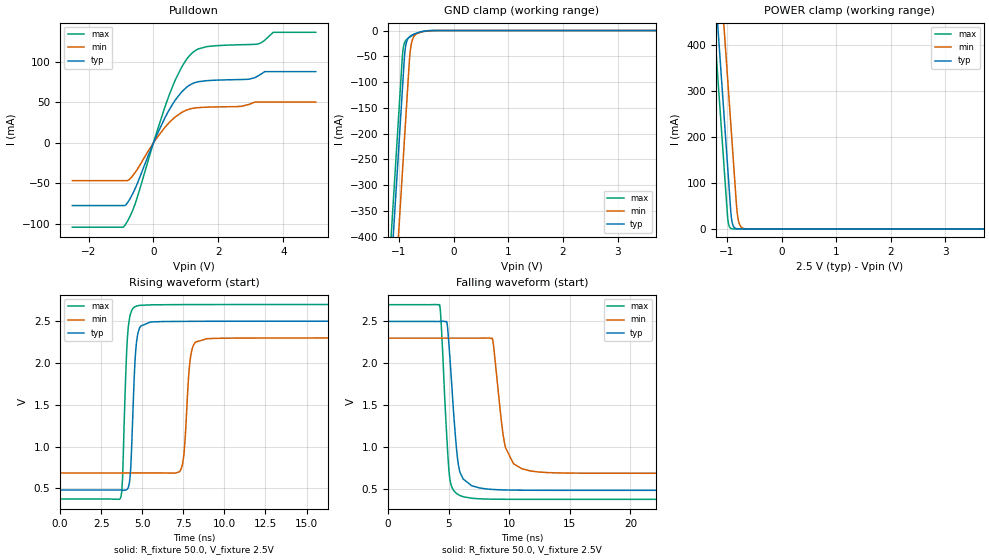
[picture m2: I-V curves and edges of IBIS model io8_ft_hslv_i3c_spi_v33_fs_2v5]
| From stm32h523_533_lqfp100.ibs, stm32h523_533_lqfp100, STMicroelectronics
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[Model]   io8_ft_hslv_i3c_spi_v33_fs_2v5
Model_type I/O_open_drain
Polarity   Non-Inverting
Enable   Active-Low
| CAP_THRESHOLD on pad IOFT is "UDTCAPC" :
| Rising=20.0% of vddiom   Falling=80.0% of vddiom
| C_comp min and max val. don't necessarily correlate with the min and max pvt
| but are the smallest and greatest pad capacitance found.
| var   typ   min   max
C_comp   3.86841pF  3.83550pF  3.96274pF
|C_comp_pulldown   3.86841pF  3.83550pF  3.96274pF
Vinl = 1.15V
Vinh = 1.35V
Vmeas = 1.25V   | Reference voltage for timing measurements
Cref  = 50.0pF   | Timing specification test load capacitance value
Rref  = 1.0MOhm   | Timing specification test load resistance value
Vref  = 1.375V   | Timing specification test load voltage
[Model Spec]
| TIME_THRESHOLD on pin ZII2CV11 is "CMOS" :
| Rising=40.0% of vdd   Falling=60.0% of vdd
Vinl 978.80000mV 906.80000mV 1.05480V
Vinh 1.39920V 1.29220V 1.48720V
| variable   typ   min   max
[Temperature Range] 25.0 125.0 -40.0
| variable   typ   min   max
[Voltage Range] 2.5V 2.3V 2.7V
| variable   typ   min   max
[POWER Clamp Reference] 2.5V 2.3V 2.7V
| variable   typ   min   max
[GND Clamp Reference] 0V 0V 0V
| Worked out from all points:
|   slope of the pulldown table from 0 to 0.375 V, typ, clamps not added: 11.5 ohm
|   GND clamp passes 1 mA (typ) near -0.52 V on its own axis
|   POWER clamp passes 1 mA (typ) near -0.84 V on its own axis
|   rising waveform, R_fixture 50.0, V_fixture 2.5V: 20-80 % time 253ps typ, 305ps min, 242ps max; typ from 0.481 V to 2.5 V
|   falling waveform, R_fixture 50.0, V_fixture 2.5V: 20-80 % time 627ps typ, 795ps min, 493ps max; typ from 2.5 V to 0.481 V
[POWER Clamp]
-2.5V     2.708A     2.899A     2.597A
-1.23V    548.8mA    740.2mA    437.5mA
-1.16V    429.8mA    621.2mA    318.5mA
-1.12V    361.8mA    553.2mA    250.5mA
-1.03V    208.8mA    400.2mA    97.53mA
-980mV    123.8mA    315.2mA    17.95mA
-920mV    26.3mA     213.2mA    906uA
-880mV    5.543mA    145.2mA    123.7uA
-810mV    363.5uA    33.6mA     3.797uA
-770mV    76.62uA    10.47mA    518.8nA
-700mV    5.026uA    1.361mA    16.09nA
5V        0A         0A         0A
[GND Clamp]
-2.5V     -2.77A     -2.931A    -2.704A
-1.21V    -576.8mA   -738.1mA   -511.3mA
-950mV    -134.8mA   -296.1mA   -69.34mA
-920mV    -83.82mA   -245.1mA   -32.48mA
-900mV    -50.56mA   -211.1mA   -24.02mA
-880mV    -31.31mA   -177.1mA   -19.85mA
-850mV    -18.7mA    -126.1mA   -16.34mA
-800mV    -11.46mA   -46.18mA   -12.45mA
-750mV    -8.203mA   -16.63mA   -9.325mA
-650mV    -4.063mA   -4.987mA   -4.427mA
-360mV    -35.05uA   -165.1uA   -9.564uA
5V        7.96nA     1.282uA    294pA
| variable   typ   min   max
[Pullup Reference] 2.5V 2.3V 2.7V
| variable   typ   min   max
[Pulldown Reference] 0V 0V 0V
[Pulldown]
-2.5V     -77.63mA   -46.85mA   -104.3mA
-870mV    -77.24mA   -46.85mA   -101.4mA
-550mV    -55.3mA    -35.88mA   -73.72mA
90mV      8.401mA    5.299mA    11.79mA
610mV     49.03mA    29.76mA    71.69mA
870mV     62.92mA    37.48mA    93.62mA
1.23V     73.63mA    42.72mA    112.2mA
1.64V     76.78mA    44.01mA    118.8mA
2.7V      78.15mA    44.99mA    121.2mA
3.22V     82.58mA    50.35mA    122.2mA
3.69V     87.93mA    50.35mA    136.5mA
5V        87.93mA    50.35mA    136.5mA
[Ramp]
dV/dt_r 1.21162V/248.59251ps 969.21784mV/300.85866ps 1.39626V/238.23524ps
dV/dt_f 1.21165V/625.63705ps 969.26011mV/793.66724ps 1.39628V/491.55772ps
R_load = 50.0
| Removed startup time: 0s 0s 0s  .
| Removed end time: 33.7ns.
[Rising Waveform]
R_fixture   = 50.0
V_fixture   = 2.5V
V_fixture_min = 2.3V
V_fixture_max = 2.7V
0s        480.6mV    684.6mV    372.9mV
3.7ns     480.5mV    684.6mV    398.6mV
3.8ns     479.7mV    684.6mV    621.4mV
4.1ns     493.9mV    684.6mV    2.318V
4.3ns     752.8mV    684.6mV    2.599V
4.65ns    2.252V     684.6mV    2.681V
7.35ns    2.498V     726.9mV    2.699V
8ns       2.498V     2.14V      2.699V
8.95ns    2.499V     2.291V     2.7V
33.7ns    2.5V       2.3V       2.7V
| Removed startup time: 0s 0s 0s  .
| Removed end time: 33.75ns.
[Falling Waveform]
R_fixture   = 50.0
V_fixture   = 2.5V
V_fixture_min = 2.3V
V_fixture_max = 2.7V
0s        2.5V       2.3V       2.7V
4.25ns    2.5V       2.3V       2.702V
4.85ns    2.494V     2.3V       1.112V
5.05ns    2.173V     2.3V       676.5mV
5.6ns     1.058V     2.3V       449.7mV
5.9ns     716.9mV    2.3V       421.3mV
8.6ns     491.4mV    2.298V     375mV
9.65ns    485.1mV    1.02V      373.7mV
11.05ns   482.1mV    737.9mV    373.1mV
33.75ns   480.6mV    684.6mV    372.9mV
